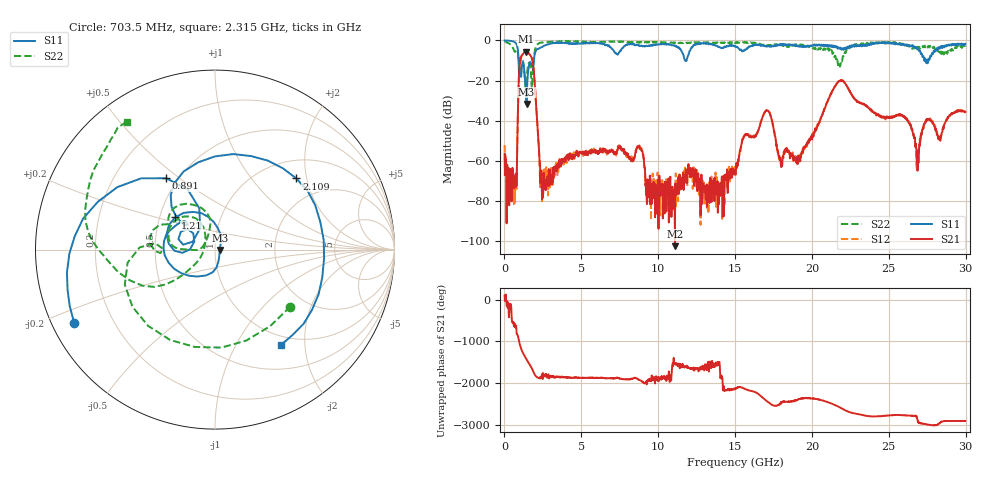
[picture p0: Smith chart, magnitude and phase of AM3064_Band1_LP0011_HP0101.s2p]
# Hz S DB R 50.0
!freq dBS11 angS11 dBS21 angS21 dBS12 angS12 dBS22 angS22
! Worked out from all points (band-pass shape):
!   1600 points, 10 MHz to 29.98 GHz, reference 50 ohm
!   highest |S21| = -5.57 dB at 1.397 GHz (marker M1); lowest = -102.4 dB at 11.09 GHz (marker M2)
!   |S21| within 3 dB of the highest: 1.073 GHz to 1.765 GHz (691.5 MHz wide, 48.7 % of centre)
!   lowest |S11| = -31.6 dB at 1.435 GHz (marker M3), VSWR 1.05, Z = 52.7 - j0.213 ohm
!   |S11| at or under -10 dB: 916.8 MHz to 1.914 GHz (997 MHz wide, 70.4 % of centre); 11.75 GHz to 11.84 GHz (88.43 MHz wide, 0.749 % of centre); 27.39164 GHz to 27.45933 GHz (67.69 MHz wide, 0.247 % of centre)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
!   |S22| runs from -24.0 to -0.3 dB; largest |S21 - S12| = 0.0063
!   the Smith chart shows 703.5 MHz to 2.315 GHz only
!   S11 on the Smith chart (normalised r, x): 703.5 MHz: 0.06, -0.24; 891 MHz: 0.43, +0.45; 1.21 GHz: 0.60, +0.23; 2.109 GHz: 1.40, +1.74; 2.315 GHz: 0.86, -1.56
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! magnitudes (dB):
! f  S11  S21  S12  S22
! 10 MHz  0.0  -56.4  -52.2  -0.3
! 703.5 MHz  -1.1  -67.4  -66.3  -5.6
! 891 MHz  -6.3  -30.2  -30.1  -7.5
! 1.21 GHz  -10.9  -6.7  -6.7  -10.5
! 1.397 GHz  -24.4  -5.6  -5.6  -21.7
! 1.435 GHz  -31.6  -5.6  -5.6  -18.7
! 1.809 GHz  -13.0  -9.7  -9.6  -20.5
! 2.109 GHz  -4.4  -38.1  -38.1  -2.3
! 2.315 GHz  -3.8  -61.2  -73.7  -1.3
! 5.015 GHz  -1.5  -56.4  -55.6  -0.7
! 8.763 GHz  -2.6  -52.4  -52.8  -1.1
! 10 GHz  -2.0  -69.4  -75.0  -0.9
! 11.09 GHz  -2.5  -102.4  -71.4  -1.0
! 15 GHz  -3.1  -65.0  -67.6  -1.3
! 17.03 GHz  -3.0  -34.7  -34.7  -2.6
! 17.97 GHz  -2.3  -61.1  -59.0  -2.1
! 19.99 GHz  -2.8  -47.6  -48.0  -3.4
! 21.83 GHz  -3.9  -20.1  -20.1  -13.1
! 25 GHz  -1.0  -38.6  -38.2  -1.0
! 26.85 GHz  -4.6  -61.4  -64.7  -3.2
! 27.49 GHz  -10.0  -39.8  -39.2  -3.3
! 29.98 GHz  -1.7  -35.5  -35.3  -3.2
